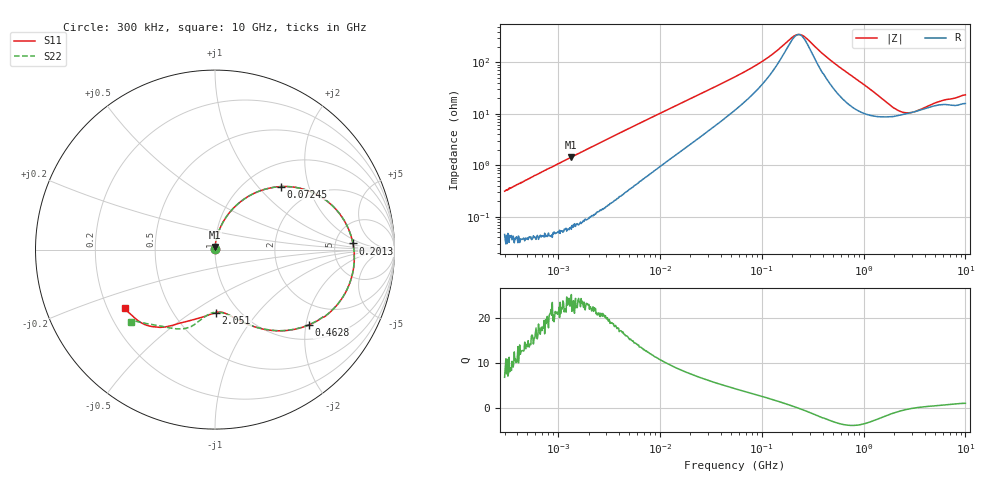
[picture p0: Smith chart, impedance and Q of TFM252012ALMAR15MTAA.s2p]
! S-Parameter Data Generated by TDK Corporation
! Copyright(C) 2019 TDK Corporation.
! All Rights Reserved.
! TDK P/N: TFM252012ALMAR15MTAA (Inductor)
! Property: L=150nH at 1MHz
! Size(LxWxT): 2.5x2x1.2mm
! Model Type: s2p (Touchstone File Format Version 1.0)
! Frequency: DC=Yes Start=0.3MHz Stop=10000MHz 802points Log-sweep
! Model Generated on May 10, 2019
! Port Assignments:
!  1 ---@@@--- 2
! Applicable Conditions:
!  Temperature = 25 degC
!  DC Bias Current = 0 A
!  Small Signal Operation
! Terms and conditions regarding TDK Simulation Models
! (1)This simulation model is being provided solely for informational purposes. Please refer to the specifications of the products in terms of detailed characteristics of such products.
! (2)In no event shall TDK Corporation of any of its subsidiaries be liable for any loss or damage arising, directly or indirectly,
!  From any information contained in this simulation model, including, but not limited to loss or damages arising from any inaccuracies, omissions or errors in connection with such information.
! (3)Any and all copyrights on this simulation model are owned by TDK Corporation.
!  Duplication or redistribution of this simulation model without prior written permission from TDK Corporation is prohibited.
! (4)This simulation model is subject to any modification or change without any prior notice.
! (5)Neither TDK Corporation nor any of its subsidiaries shall make any warranty, express or implied,
!  Including but not limited to the correctness, implied warranties of merchantability and fitness for a particular purpose with respect to this simulation models.
! (6)The use of this simulation model shall be deemed to have consented to the terms and conditions hereof.
# Hz S MA R 50
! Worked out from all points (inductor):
!   801 points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, 300 kHz to 10 GHz, reference 50 ohm
!   read as one part in series: L = 167 nH near 318.3 kHz
!   highest Q = 24 at 1.356 MHz (marker M1), where L = 169 nH
!   self-resonance near 229.6 MHz
!   S11 on the Smith chart (normalised r, x): 300 kHz: 1.00, +0.01; 72.45 MHz: 1.42, +1.35; 201.3 MHz: 7.46, +1.26; 462.8 MHz: 1.36, -2.07; 2.051 GHz: 0.79, -0.63; 10 GHz: 0.27, -0.28
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300000  0.002967 85.1  0.9995 -0.2  0.9992 -0.2  0.003181 85.8
1355528  0.01417 86.8  0.9994 -0.8  0.9993 -0.8  0.01427 86.9
1713600  0.01795 86.5  0.9991 -1.1  0.999 -1.0  0.01799 86.5
9671944  0.09605 79.1  0.9866 -5.6  0.9867 -5.6  0.09603 79.1
2.630692e7  0.2366 67.3  0.9364 -13.9  0.9364 -13.9  0.2366 67.3
5.477226e7  0.4223 51.7  0.8153 -25.1  0.8153 -25.1  0.4222 51.7
7.244865e7  0.5095 43.6  0.7319 -30.5  0.7319 -30.5  0.5094 43.6
1.210198e8  0.6685 25.2  0.5067 -38.9  0.5067 -38.9  0.6684 25.2
2.013356e8  0.7694 2.6  0.2472 -21.6  0.2472 -21.6  0.7692 2.7
2.444933e8  0.779 -7.0  0.2258 6.5  0.2259 6.5  0.7788 -6.8
3.126428e8  0.7624 -19.5  0.323 30.9  0.3231 30.9  0.7622 -19.4
4.627802e8  0.6697 -38.9  0.5523 32.0  0.5524 32.0  0.6699 -38.7
6.325141e8  0.5656 -53.1  0.6998 23.4  0.6998 23.4  0.5661 -52.9
9.101824e8  0.4508 -66.8  0.8041 11.8  0.8041 11.8  0.4516 -66.6
1.260284e9  0.3792 -76.7  0.8473 1.5  0.8473 1.5  0.3804 -76.6
1.767019e9  0.3488 -86.0  0.8569 -9.2  0.857 -9.2  0.3502 -86.7
2.051294e9  0.352 -89.1  0.8529 -13.9  0.8529 -13.9  0.3507 -91.6
3.177248e9  0.3964 -104.4  0.8085 -28.7  0.8086 -28.7  0.4045 -102.2
5.21579e9  0.4813 -119.0  0.7194 -47.4  0.7194 -47.4  0.492 -116.3
6.737565e9  0.5439 -127.5  0.6576 -59.9  0.6576 -59.9  0.544 -129.8
7.987505e9  0.5835 -137.2  0.6073 -70.0  0.6074 -70.1  0.5936 -137.7
1e10  0.598 -146.9  0.5485 -82.1  0.5487 -82.2  0.619 -139.3
